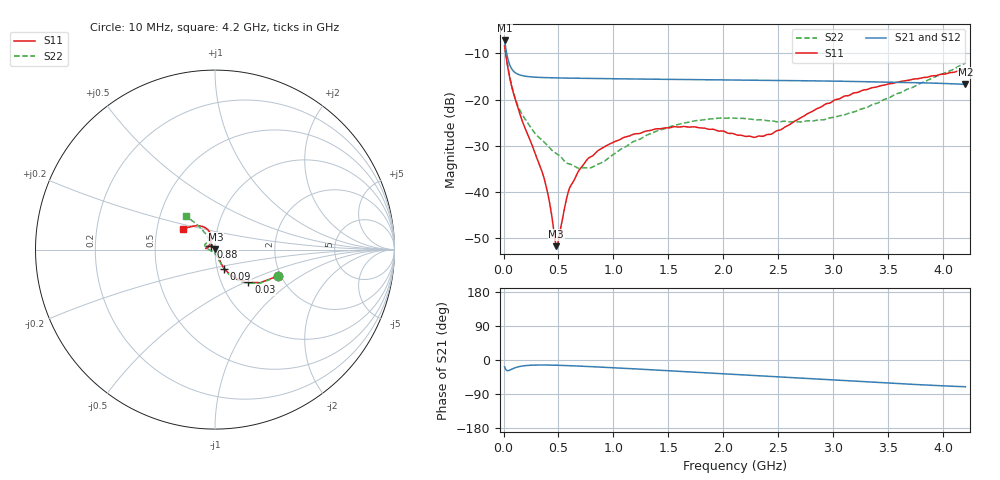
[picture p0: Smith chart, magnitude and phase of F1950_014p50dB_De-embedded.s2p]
! Integrated Device Technology
! Corporate Headquarters
! 6024 Silver Creek Valley Road
! San Jose, CA 95138  USA
! Phone:  1-408-284-8200
! Toll Free:  1-800-223-1366
! Webpage:  http://www.idt.com/
! Timing and RF Division
! 515 Groton Road, Suite 102
! Westford, MA 01886-6024
! Device:  F1950
! Description: 7-bit 0.25 dB Digital Step Attenuator
! Frequency:  150.0 -  4000.00 MHz
! Package:  4x4 mm Thin QFN Plastic Package: 24 pin
! Ports:  2 RF, 12 DC
!  Pin  1  = D0
!  Pin  2  = VDD
!  Pin  3  = Vmode
!  Pin  4  = GND
!  Pin  5  = RF1  =  Port 1
!  Pin  6  = GND
!  Pin  7  = GND
!  Pin  8  = GND
!  Pin  9  = GND
!  Pin 10  = GND
!  Pin 11  = GND
!  Pin 12  = GND
!  Pin 13  = GND
!  Pin 14  = RF2  =  Port 2
!  Pin 15  = GND
!  Pin 16  = LE
!  Pin 17  = CLK
!  Pin 18  = DATE
!  Pin 19  = D6
!  Pin 20  = D5
!  Pin 21  = D4
!  Pin 22  = D3
!  Pin 23  = D2
!  Pin 24  = D1
! State:  58
! Atten State:  14.50 dB
! Voltage:  +5.00 Volts
! Current:  Not Measured mA
! Data:  The device was measured on a the F195X evaluation board which has
!  individual transmission lines to the RF pins.  Data was collected
!  using a calibrated network analyzer.  The evaluation board was
!  de-embedded using a TRL calibration technique.
!  The reference plane is the edge of the package pin.
! Misc:  Board 2019
!  Action Tracker AT0250
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# GHz S dB R 50
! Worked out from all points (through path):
!   420 points, 10 MHz to 4.2 GHz, reference 50 ohm
!   highest |S21| = -7.19 dB at 10 MHz (marker M1); lowest = -16.7 dB at 4.2 GHz (marker M2)
!   group delay of S21, straight-line fit = 41 ps
!   lowest |S11| = -51.8 dB at 480 MHz (marker M3), VSWR 1.01, Z = 50.2 + j0.132 ohm
!   |S11| at or under -10 dB: 19.53 MHz to end of sweep
!   |S22| runs from -34.9 to -8.4 dB; largest |S21 - S12| = 0.00025
!   S11 on the Smith chart (normalised r, x): 10 MHz: 1.94, -0.66; 30 MHz: 1.34, -0.52; 90 MHz: 1.08, -0.23; 880 MHz: 0.95, +0.03; 4.2 GHz: 0.68, +0.16
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0.01  -8.37 -22.5  -7.19 -18.1  -7.19 -18.1  -8.36 -23.1
0.03  -11.68 -44.5  -10.13 -27.8  -10.13 -27.8  -11.58 -45.4
0.05  -14.50 -54.9  -12.05 -27.5  -12.05 -27.5  -14.26 -56.1
0.09  -18.61 -64.1  -13.84 -22.3  -13.84 -22.3  -18.45 -63.8
0.18  -25.26 -64.6  -14.87 -15.5  -14.87 -15.5  -23.62 -70.0
0.36  -36.36 -50.4  -15.24 -13.2  -15.24 -13.2  -29.01 -76.0
0.41  -41.26 -42.9  -15.27 -13.4  -15.27 -13.4  -30.22 -77.1
0.46  -49.00 -10.4  -15.30 -13.7  -15.30 -13.7  -31.39 -82.7
0.48  -51.79 30.8  -15.31 -13.8  -15.31 -13.8  -31.70 -85.1
0.5  -50.42 73.9  -15.32 -14.0  -15.32 -14.0  -32.00 -86.6
0.59  -39.97 119.6  -15.36 -14.9  -15.36 -14.9  -33.90 -98.7
0.71  -34.63 131.4  -15.40 -16.4  -15.40 -16.4  -34.84 -119.2
0.88  -30.79 142.0  -15.45 -18.7  -15.45 -18.8  -33.81 -151.0
1.1  -28.18 153.5  -15.52 -22.0  -15.52 -22.0  -30.34 -175.4
1.41  -26.35 166.3  -15.60 -26.8  -15.60 -26.8  -26.68 170.1
1.73  -25.91 173.0  -15.68 -31.8  -15.67 -31.9  -24.65 161.1
2.11  -27.58 163.8  -15.77 -38.1  -15.77 -38.1  -24.07 151.8
2.43  -27.54 130.3  -15.85 -43.3  -15.85 -43.3  -24.60 142.4
2.81  -22.55 107.0  -15.95 -49.7  -15.95 -49.7  -24.65 127.6
3.11  -19.21 109.1  -16.05 -54.7  -16.05 -54.7  -23.24 121.4
3.51  -16.59 119.1  -16.22 -61.1  -16.21 -61.1  -19.61 120.8
4.2  -13.36 147.3  -16.71 -70.6  -16.70 -70.6  -12.10 130.5
